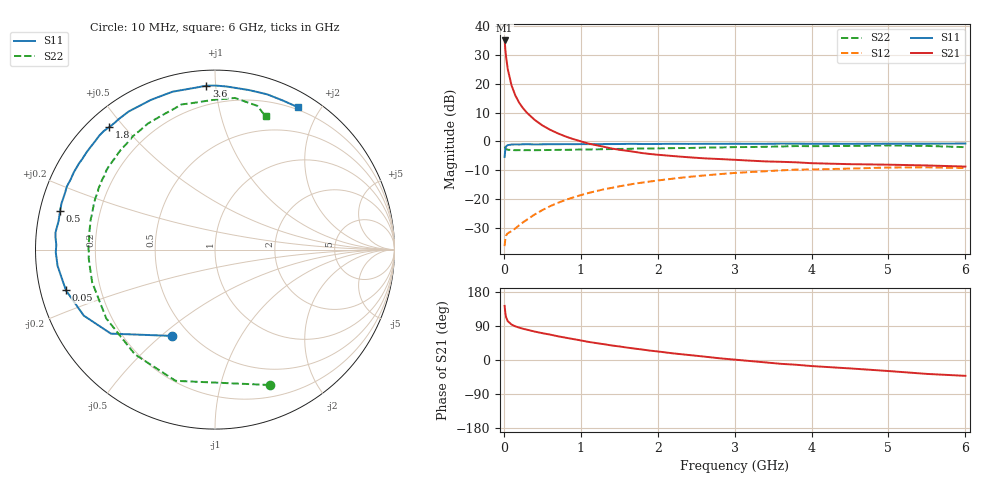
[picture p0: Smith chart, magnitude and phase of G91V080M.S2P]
! SIEMENS Small Signal Semiconductors
! BFG235
! Si NPN RF Bipolar Junction Transistor in SOT223
! VCE = 1 V  IC = 80 mA
! Common Emitter S-Parameters:  July  1994
# GHz  S  MA  R  50
!  f  S11  S21  S12  S22
! GHz  MAG  ANG  MAG  ANG  MAG  ANG  MAG  ANG
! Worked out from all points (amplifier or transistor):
!   40 points, 10 MHz to 6 GHz, reference 50 ohm
!   highest |S21| = 35.0 dB at 10 MHz (marker M1)
!   |S21| within 3 dB of that: start of sweep to 19.48 MHz
!   unconditionally stable (mu >= 1): 428.6 MHz to 1.676 GHz; 1.715 GHz to 1.991 GHz
!   at 200 MHz: K = 0.77, MSG = 21.2 dB, |S12| = -29.0 dB
!   at 1.5 GHz: K = 1.03, MAG = 5.4 dB, |S12| = -15.6 dB
!   at 6 GHz: K = 0.95, MSG = 0.3 dB, |S12| = -9.2 dB
!   S11 on the Smith chart (normalised r, x): 10 MHz: 0.40, -0.54; 50 MHz: 0.08, -0.13; 500 MHz: 0.06, +0.12; 1.8 GHz: 0.06, +0.46; 3.6 GHz: 0.08, +0.95; 6 GHz: 0.17, +1.73
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0.01  0.5373 -116.5  56.06 142.9  0.0153 54.3  0.8137 -68.0
0.02  0.7456 -141.1  38.95 123.1  0.021 38.1  0.7634 -106.7
0.03  0.8185 -153.3  28.56 112.6  0.0236 31.2  0.7347 -127.4
0.05  0.861 -164.7  18.13 102.8  0.0255 26.2  0.717 -147.7
0.1  0.8818 -174.1  9.321 93.6  0.0279 30.1  0.7082 -165.1
0.15  0.8873 -179.0  6.225 88.7  0.0311 37.0  0.7038 -172.2
0.2  0.8845 178.3  4.656 85.4  0.0353 42.0  0.7053 -176.1
0.25  0.8907 175.8  3.749 82.4  0.0397 45.7  0.7035 -179.0
0.3  0.8937 173.9  3.135 80.0  0.044 49.3  0.7054 178.5
0.4  0.8858 169.6  2.362 75.1  0.0541 53.0  0.7038 174.9
0.5  0.8895 166.1  1.895 70.8  0.0645 55.0  0.7068 171.8
0.7  0.893 159.5  1.382 62.7  0.0859 56.1  0.7128 166.2
0.9  0.8942 154.2  1.099 55.3  0.1067 54.3  0.7175 161.3
1.1  0.8969 147.8  0.917 47.8  0.1276 51.9  0.7259 156.6
1.4  0.8985 140.6  0.754 38.4  0.1566 47.0  0.7363 150.0
1.8  0.9013 130.8  0.627 27.6  0.1934 40.0  0.7521 141.7
2.2  0.9074 122.0  0.557 17.5  0.2263 32.5  0.7645 133.5
3.2  0.9075 100.9  0.464 -2.7  0.2942 13.2  0.7988 114.6
3.6  0.9148 93.0  0.443 -10.1  0.3144 4.9  0.8163 106.4
4.5  0.9088 77.9  0.403 -22.2  0.3379 -10.5  0.8339 90.9
5.5  0.9127 65.2  0.383 -36.7  0.3555 -27.9  0.8348 73.6
6  0.9179 59.8  0.366 -41.8  0.3449 -34.4  0.7941 69.2
